| TEXAS INSTRUMENTS INCORPORATED
| Standard Linear and Logic Group
| IBIS Model of SN74LVT245B
| 3.3-V ABT OCTAL BUS TRANSCEIVER WITH 3-STATE OUTPUTS
| This file contains package information for the following:
|  QFN 20-pin (RGY) package as [Component] LVT245M_RGY
|  SOIC 20-pin (DW) package as [Component] LVT245M_DW
|  SOP 20-pin (NS) package as [Component] LVT245M_NS
|  SSOP 20-pin (DB) package as [Component] LVT245M_DB
|  TSSOP 20-pin (PW) package as [Component] LVT245M_PW
|  jrBGA 20-pin (GQN) package as [Component] LVT245M_GQN
|  jrBGA 20-pin (ZQN) package as [Component] LVT245M_ZQN
| This device can be powered at the following Vccs:
|  3.3 volt Vcc
| This file provides unique models under the [Model Selector] for each Vcc.
| For operation at a specific Vcc, select the appropriate model after each
| [Model Selector] keyword.
[IBIS Ver]   3.2
[Comment char]  |_char
[File Name]   sn74lvt245b.ibs
[File Rev]   2.3 | m_die
[Date]   May 15, 2007
[Source]   Data created from TI-SPICE simulations at TI-SLL.
[Notes]   The following is an IBIS list for the SN74LVT245B.
   Please contact sllibis@ti.com with questions and
   comments concerning SLL IBIS models.
   - FILE REV HISTORY
   - 2.3 Release New creation of IBIS file on 6/6/2007
   - Power clamp data deleted as there is no power-clamp diode.
[Disclaimer] Property of Texas Instruments Incorporated.  Unauthorized
   reproduction and/or distribution is strictly prohibited.
   This product is protected under copyright law.
   Created  2007, (C) Copyright  2007, Texas Instruments
   Incorporated, All Rights Reserved
   UNLESS THERE IS A SIGNED, WRITTEN AGREEMENT TO THE
   CONTRARY, TEXAS INSTRUMENTS (TI) IS PROVIDING THE IBIS
   MODELS  AND WITHOUT ANY WARRANTY, EXPRESSED OR
   IMPLIED.  TI assumes no liability for:
   1) the accuracy of the IBIS models provided to your
   company;
   2) the proper functioning of these IBIS Models in your
   design or for any resulting applications; or
   3) infringement of patents, copyrights or intellectual
   property rights resulting from your use of these IBIS
   models.
   TI provides IBIS Models as a service to our customers.
   You and your company shall not distribute, sell or give
   these models to anyone else without prior written
   permission from TI.
   TI reserves the right to make changes to our products or
   to discontinue any semiconductor product or service
   without notice, and advises our customers to obtain the
   latest version of relevant information to verify, before
   placing orders, that the information being relied on is
   current.
   Please be aware that your receipt and use of the IBIS
   information provided shall serve as acceptance of these
   terms and conditions.  If you do not accept these terms,
   you should return or destroy the IBIS models and any
   other accompanying information immediately.
| Component SN74LVT245B_RGY 20-PIN QFN
[Component]   SN74LVT245B_RGY
[Manufacturer]   Texas Instruments, Inc.
[Package]
|   typ   min   max
R_pkg   5.000e-02   4.600e-02   5.500e-02
L_pkg   1.119e-09   1.025e-09   1.227e-09
C_pkg   3.520e-13   3.440e-13   3.630e-13
[Pin]   signal_name   model_name   R_pin   L_pin   C_pin
1   DIR   LVT245_INDIR   5.200e-02   1.167e-09   3.600e-13
2   A1   LVT245_IO   4.700e-02   1.049e-09   3.440e-13
3   A2   LVT245_IO   4.700e-02   1.055e-09   3.450e-13
4   A3   LVT245_IO   5.000e-02   1.119e-09   3.500e-13
5   A4   LVT245_IO   5.500e-02   1.227e-09   3.600e-13
6   A5   LVT245_IO   5.200e-02   1.167e-09   3.550e-13
7   A6   LVT245_IO   4.900e-02   1.087e-09   3.480e-13
8   A7   LVT245_IO   4.700e-02   1.054e-09   3.460e-13
9   A8   LVT245_IO   4.900e-02   1.091e-09   3.490e-13
10   GND   GND   5.300e-02   1.184e-09   3.620e-13
11   B8   LVT245_IO   5.300e-02   1.181e-09   3.600e-13
12   B7   LVT245_IO   5.000e-02   1.108e-09   3.490e-13
13   B6   LVT245_IO   4.800e-02   1.075e-09   3.470e-13
14   B5   LVT245_IO   5.000e-02   1.107e-09   3.490e-13
15   B4   LVT245_IO   5.400e-02   1.200e-09   3.620e-13
16   B3   LVT245_IO   5.100e-02   1.141e-09   3.570e-13
17   B2   LVT245_IO   4.700e-02   1.043e-09   3.440e-13
18   B1   LVT245_IO   4.600e-02   1.025e-09   3.440e-13
19   NOE   LVT245_INNOE   4.900e-02   1.090e-09   3.490e-13
20   VCC   POWER   5.400e-02   1.204e-09   3.630e-13
| Component SN74LVT245B_DW 20-PIN SOIC
[Component]   SN74LVT245B_DW
[Manufacturer]   Texas Instruments, Inc.
[Package]
|   typ   min   max
R_pkg   3.800e-02   3.300e-02   4.500e-02
L_pkg   5.012e-09   4.110e-09   6.349e-09
C_pkg   7.170e-13   5.300e-13   8.680e-13
[Pin]   signal_name   model_name   R_pin   L_pin   C_pin
1   DIR   LVT245_INDIR   4.200e-02   6.336e-09   8.650e-13
2   A1   LVT245_IO   4.300e-02   5.542e-09   8.670e-13
3   A2   LVT245_IO   3.400e-02   4.714e-09   7.320e-13
4   A3   LVT245_IO   3.400e-02   4.377e-09   5.910e-13
5   A4   LVT245_IO   3.600e-02   4.130e-09   5.330e-13
6   A5   LVT245_IO   3.500e-02   4.111e-09   5.300e-13
7   A6   LVT245_IO   3.400e-02   4.284e-09   5.830e-13
8   A7   LVT245_IO   3.400e-02   4.634e-09   7.260e-13
9   A8   LVT245_IO   4.000e-02   5.518e-09   8.650e-13
10   GND   GND   4.300e-02   6.349e-09   8.660e-13
11   B8   LVT245_IO   4.100e-02   6.281e-09   8.610e-13
12   B7   LVT245_IO   4.500e-02   5.561e-09   8.680e-13
13   B6   LVT245_IO   3.300e-02   4.778e-09   7.420e-13
14   B5   LVT245_IO   3.500e-02   4.414e-09   5.960e-13
15   B4   LVT245_IO   3.500e-02   4.110e-09   5.330e-13
16   B3   LVT245_IO   3.600e-02   4.130e-09   5.330e-13
17   B2   LVT245_IO   3.400e-02   4.377e-09   5.910e-13
18   B1   LVT245_IO   3.400e-02   4.714e-09   7.310e-13
19   NOE   LVT245_INNOE   4.300e-02   5.569e-09   8.680e-13
20   VCC   POWER   4.200e-02   6.308e-09   8.640e-13
| Component SN74LVT245B_NS 20-PIN SOP
[Component]   SN74LVT245B_NS
[Manufacturer]   Texas Instruments, Inc.
[Package]
|   typ   min   max
R_pkg   4.400e-02   2.900e-02   5.800e-02
L_pkg   3.666e-09   2.317e-09   5.115e-09
C_pkg   5.480e-13   3.160e-13   7.250e-13
[Pin]   signal_name   model_name   R_pin   L_pin   C_pin
1   DIR   LVT245_INDIR   5.800e-02   5.115e-09   7.250e-13
2   A1   LVT245_IO   5.300e-02   4.591e-09   7.240e-13
3   A2   LVT245_IO   4.900e-02   3.754e-09   5.720e-13
4   A3   LVT245_IO   2.900e-02   2.549e-09   3.880e-13
5   A4   LVT245_IO   3.100e-02   2.317e-09   3.160e-13
6   A5   LVT245_IO   3.100e-02   2.317e-09   3.160e-13
7   A6   LVT245_IO   2.900e-02   2.556e-09   3.990e-13
8   A7   LVT245_IO   4.900e-02   3.754e-09   5.790e-13
9   A8   LVT245_IO   5.300e-02   4.591e-09   7.240e-13
10   GND   GND   5.800e-02   5.115e-09   7.250e-13
11   B8   LVT245_IO   5.800e-02   5.115e-09   7.250e-13
12   B7   LVT245_IO   5.300e-02   4.591e-09   7.240e-13
13   B6   LVT245_IO   4.900e-02   3.754e-09   5.790e-13
14   B5   LVT245_IO   2.900e-02   2.557e-09   3.990e-13
15   B4   LVT245_IO   3.100e-02   2.317e-09   3.160e-13
16   B3   LVT245_IO   3.100e-02   2.317e-09   3.160e-13
17   B2   LVT245_IO   2.900e-02   2.557e-09   3.990e-13
18   B1   LVT245_IO   4.900e-02   3.754e-09   5.790e-13
19   NOE   LVT245_INNOE   5.300e-02   4.591e-09   7.240e-13
20   VCC   POWER   5.800e-02   5.115e-09   7.250e-13
| Component SN74LVT245B_DB 20-PIN SSOP
[Component]   SN74LVT245B_DB
[Manufacturer]   Texas Instruments, Inc.
[Package]
|   typ   min   max
R_pkg   4.000e-02   3.500e-02   5.100e-02
L_pkg   3.495e-09   3.035e-09   4.314e-09
C_pkg   4.200e-13   3.460e-13   5.020e-13
[Pin]   signal_name   model_name   R_pin   L_pin   C_pin
1   DIR   LVT245_INDIR   4.900e-02   4.310e-09   5.020e-13
2   A1   LVT245_IO   4.800e-02   3.903e-09   4.870e-13
3   A2   LVT245_IO   3.500e-02   3.189e-09   3.960e-13
4   A3   LVT245_IO   3.500e-02   3.036e-09   3.470e-13
5   A4   LVT245_IO   3.500e-02   3.035e-09   3.670e-13
6   A5   LVT245_IO   3.500e-02   3.035e-09   3.670e-13
7   A6   LVT245_IO   3.500e-02   3.036e-09   3.470e-13
8   A7   LVT245_IO   3.500e-02   3.189e-09   3.970e-13
9   A8   LVT245_IO   4.700e-02   3.899e-09   4.880e-13
10   GND   GND   5.100e-02   4.314e-09   5.000e-13
11   B8   LVT245_IO   5.100e-02   4.314e-09   5.000e-13
12   B7   LVT245_IO   4.700e-02   3.899e-09   4.880e-13
13   B6   LVT245_IO   3.500e-02   3.189e-09   3.970e-13
14   B5   LVT245_IO   3.500e-02   3.036e-09   3.460e-13
15   B4   LVT245_IO   3.500e-02   3.035e-09   3.670e-13
16   B3   LVT245_IO   3.500e-02   3.035e-09   3.670e-13
17   B2   LVT245_IO   3.500e-02   3.036e-09   3.460e-13
18   B1   LVT245_IO   3.500e-02   3.189e-09   3.970e-13
19   NOE   LVT245_INNOE   4.700e-02   3.899e-09   4.880e-13
20   VCC   POWER   5.100e-02   4.314e-09   5.020e-13
| Component SN74LVT245B_PW 20-PIN TSSOP
[Component]   SN74LVT245B_PW
[Manufacturer]   Texas Instruments, Inc.
[Package]
|   typ   min   max
R_pkg   5.000e-02   4.200e-02   6.000e-02
L_pkg   2.802e-09   2.248e-09   3.553e-09
C_pkg   3.170e-13   2.020e-13   4.430e-13
[Pin]   signal_name   model_name   R_pin   L_pin   C_pin
1   DIR   LVT245_INDIR   5.500e-02   3.461e-09   4.400e-13
2   A1   LVT245_IO   5.500e-02   3.150e-09   4.010e-13
3   A2   LVT245_IO   4.200e-02   2.619e-09   3.020e-13
4   A3   LVT245_IO   4.500e-02   2.273e-09   2.020e-13
5   A4   LVT245_IO   4.500e-02   2.248e-09   2.240e-13
6   A5   LVT245_IO   4.500e-02   2.273e-09   2.260e-13
7   A6   LVT245_IO   4.400e-02   2.323e-09   2.050e-13
8   A7   LVT245_IO   4.600e-02   2.704e-09   3.070e-13
9   A8   LVT245_IO   6.000e-02   3.265e-09   4.110e-13
10   GND   GND   5.700e-02   3.506e-09   4.360e-13
11   B8   LVT245_IO   5.800e-02   3.553e-09   4.370e-13
12   B7   LVT245_IO   5.800e-02   3.193e-09   4.050e-13
13   B6   LVT245_IO   4.200e-02   2.704e-09   3.110e-13
14   B5   LVT245_IO   4.600e-02   2.392e-09   2.100e-13
15   B4   LVT245_IO   4.700e-02   2.334e-09   2.290e-13
16   B3   LVT245_IO   4.700e-02   2.300e-09   2.270e-13
17   B2   LVT245_IO   4.700e-02   2.349e-09   2.070e-13
18   B1   LVT245_IO   4.500e-02   2.677e-09   3.060e-13
19   NOE   LVT245_INNOE   6.000e-02   3.235e-09   4.060e-13
20   VCC   POWER   5.600e-02   3.487e-09   4.430e-13
| Component SN74LVT245B_GQN 20-PIN JRBGA
[Component]   SN74LVT245B_GQN
[Manufacturer]   Texas Instruments, Inc.
[Package]
|   typ   min   max
R_pkg   4.300e-02   3.300e-02   6.100e-02
L_pkg   1.317e-09   8.960e-10   2.088e-09
C_pkg   1.130e-13   6.400e-14   1.900e-13
[Pin]   signal_name   model_name   R_pin   L_pin   C_pin
1   DIR   LVT245_INDIR   3.800e-02   1.199e-09   1.210e-13
2   A1   LVT245_IO   4.000e-02   1.067e-09   1.020e-13
3   A2   LVT245_IO   6.100e-02   1.999e-09   1.900e-13
4   A3   LVT245_IO   3.300e-02   9.630e-10   7.100e-14
5   A4   LVT245_IO   4.900e-02   1.523e-09   1.230e-13
6   A5   LVT245_IO   3.300e-02   8.960e-10   6.400e-14
7   A6   LVT245_IO   6.100e-02   1.899e-09   1.640e-13
8   A7   LVT245_IO   3.300e-02   8.980e-10   6.700e-14
9   A8   LVT245_IO   4.900e-02   1.514e-09   1.280e-13
10   GND   GND   3.600e-02   1.006e-09   9.400e-14
11   B8   LVT245_IO   4.900e-02   1.683e-09   1.460e-13
12   B7   LVT245_IO   3.300e-02   1.121e-09   8.900e-14
13   B6   LVT245_IO   6.100e-02   2.088e-09   1.730e-13
14   B5   LVT245_IO   3.300e-02   1.027e-09   7.100e-14
15   B4   LVT245_IO   4.900e-02   1.558e-09   1.240e-13
16   B3   LVT245_IO   3.300e-02   9.280e-10   6.700e-14
17   B2   LVT245_IO   6.100e-02   1.921e-09   1.770e-13
18   B1   LVT245_IO   3.300e-02   9.010e-10   7.700e-14
19   NOE   LVT245_INNOE   3.700e-02   9.900e-10   9.800e-14
20   VCC   POWER   3.500e-02   1.168e-09   1.190e-13
| Component SN74LVT245B_ZQN 20-PIN JRBGA
[Component]   SN74LVT245B_ZQN
[Manufacturer]   Texas Instruments, Inc.
[Package]
|   typ   min   max
R_pkg   4.300e-02   3.300e-02   6.100e-02
L_pkg   1.317e-09   8.960e-10   2.088e-09
C_pkg   1.130e-13   6.400e-14   1.900e-13
[Pin]   signal_name   model_name   R_pin   L_pin   C_pin
1   DIR   LVT245_INDIR   3.800e-02   1.199e-09   1.210e-13
2   A1   LVT245_IO   4.000e-02   1.067e-09   1.020e-13
3   A2   LVT245_IO   6.100e-02   1.999e-09   1.900e-13
4   A3   LVT245_IO   3.300e-02   9.630e-10   7.100e-14
5   A4   LVT245_IO   4.900e-02   1.523e-09   1.230e-13
6   A5   LVT245_IO   3.300e-02   8.960e-10   6.400e-14
7   A6   LVT245_IO   6.100e-02   1.899e-09   1.640e-13
8   A7   LVT245_IO   3.300e-02   8.980e-10   6.700e-14
9   A8   LVT245_IO   4.900e-02   1.514e-09   1.280e-13
10   GND   GND   3.600e-02   1.006e-09   9.400e-14
11   B8   LVT245_IO   4.900e-02   1.683e-09   1.460e-13
12   B7   LVT245_IO   3.300e-02   1.121e-09   8.900e-14
13   B6   LVT245_IO   6.100e-02   2.088e-09   1.730e-13
14   B5   LVT245_IO   3.300e-02   1.027e-09   7.100e-14
15   B4   LVT245_IO   4.900e-02   1.558e-09   1.240e-13
16   B3   LVT245_IO   3.300e-02   9.280e-10   6.700e-14
17   B2   LVT245_IO   6.100e-02   1.921e-09   1.770e-13
18   B1   LVT245_IO   3.300e-02   9.010e-10   7.700e-14
19   NOE   LVT245_INNOE   3.700e-02   9.900e-10   9.800e-14
20   VCC   POWER   3.500e-02   1.168e-09   1.190e-13
| Models and submodels in the file (3): LVT245_INNOE (Input), LVT245_INDIR (Input), LVT245_IO (3-state)
